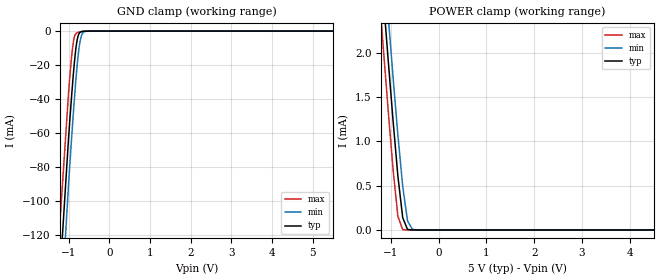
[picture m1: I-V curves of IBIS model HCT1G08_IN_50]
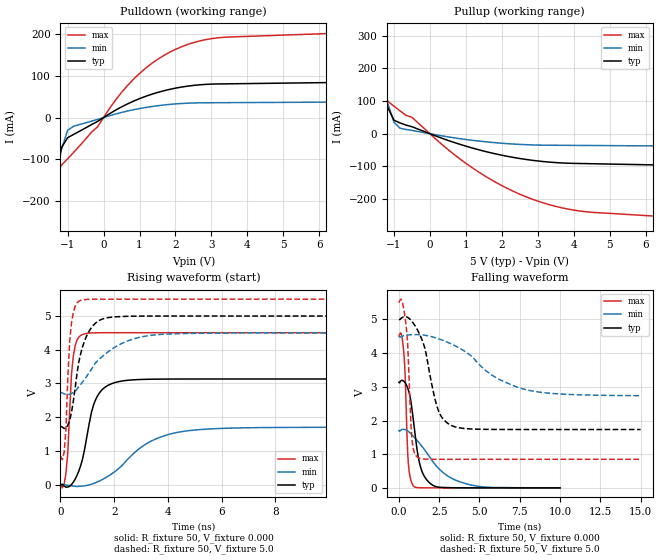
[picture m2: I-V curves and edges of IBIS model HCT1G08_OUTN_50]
| NXP Semiconductors
| Logic Products Group
| IBIS model of 74HCT1G08
| 5V 2-INPUT AND GATE
|[Packages]:
|[Package1]: TSSOP5 (GW) 5-pins Package
|[Package2]: TSSOP5 (GV) 5-pins Package
[IBIS Ver]   3.2
[File Name]   hct1g08.ibs
[File Rev]   1.0
[Date]   07-Nov-2012
[Source]   File created from simulations by LPG
   NXP Semiconductors Nijmegen
[Notes]   V1.0   Ibis model.
   Revision History
   Version Date   Author/Editor  Description
   1.0   November 2012  RRV   Initial Model
   Remarks: - IBISCHK 5.1.0 used
[Disclaimer]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
[Copyright]
   (C) Copyright 2012 NXP Semiconductors
   All rights reserved
|   Info for  TSSOP5 (GW) 5-pins Package
[Component]   74HCT1G08_GW
[Manufacturer]   NXP Semiconductors
[Package]
|   Typ   Min   Max
R_pkg   8.353E-02   8.341E-02   8.366E-02
L_pkg   1.484E-09   1.480E-09   1.486E-09
C_pkg   2.355E-13   1.892E-13   3.527E-13
[Pin] signal_name   model_name   R_pin   L_pin   C_pin
   1   B   HCT1G08_IN_50 8.357E-02 1.485E-09 2.132E-13
   2   A   HCT1G08_IN_50 8.366E-02 1.480E-09 2.311E-13
   3   GND   GND 8.354E-02 1.484E-09 1.914E-13
   4   Y   HCT1G08_OUTN_50 8.351E-02 1.486E-09 1.892E-13
   5   VCC   POWER 8.341E-02 1.486E-09 3.527E-13
|   Info for  TSSOP5 (GV) 5-pins Package
[Component]   74HCT1G08_GV
[Manufacturer]   NXP Semiconductors
[Package]
|   Typ   Min   Max
R_pkg   8.192E-02   8.186E-02   8.199E-02
L_pkg   1.305E-09   1.300E-09   1.309E-09
C_pkg   2.711E-13   2.208E-13   4.174E-13
[Pin] signal_name   model_name   R_pin   L_pin   C_pin
   1   B   HCT1G08_IN_50 8.195E-02 1.309E-09 2.208E-13
   2   A   HCT1G08_IN_50 8.199E-02 1.307E-09 2.559E-13
   3   GND   GND 8.194E-02 1.309E-09 4.174E-13
   4   Y   HCT1G08_OUTN_50 8.188E-02 1.300E-09 2.377E-13
   5   VCC   POWER 8.186E-02 1.300E-09 2.239E-13
| Models and submodels in the file (2): HCT1G08_IN_50 (Input), HCT1G08_OUTN_50 (Output)
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|   Model HCT1G08_IN_50
[Model]   HCT1G08_IN_50
Model_type   Input
Vinl = 0.8V
Vinh = 2.0V
C_comp   2.8774pF   1.2578pF   5.2328pF
[Model Spec]
| Note: The input and output voltage ratings may be exceeded if the input and
|   output current ratings are observed (please refer to the data sheet)
|   Subparameter   typ   min   max
| Thresholds
Vinl   0.8   0.8   0.8
Vinh   2.0   2.0   2.0
| Overshoot
S_overshoot_high   7.0   7.0   7.0
S_overshoot_low   -0.5   -0.5   -0.5
D_overshoot_high   7.2   7.2   7.2
D_overshoot_low   -1.3   -1.3   -1.3
D_overshoot_time   3n   3n   3n
|Ambient temperature:   25   85   -40
[Temperature Range]   35   95   -30
[Voltage Range]   5.0   4.5   5.5
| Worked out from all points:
|   GND clamp passes 1 mA (typ) near -0.73 V on its own axis
|   POWER clamp passes 1 mA (typ) near -0.92 V on its own axis
|Process Range   nominal   slow   fast
[GND_clamp]
|   voltage   I(typ)   I(min)   I(max)
-5.5V     -1.839A    -1.974A    -1.717A
-1.9V     -405mA     -453.2mA   -359.4mA
-1V       -62.81mA   -90.06mA   -36.07mA
-937.5mV  -42.01mA   -67.28mA   -18.13mA
-887.5mV  -26.77mA   -49.95mA   -7.313mA
-837.5mV  -13.86mA   -33.87mA   -2.148mA
-787.5mV  -5.045mA   -19.81mA   -915.9uA
-737.5mV  -1.287mA   -9.108mA   -551.9uA
-700mV    -465.6uA   -4.104mA   -378.7uA
-650mV    -161.3uA   -1.11mA    -204.8uA
-575mV    -48.51uA   -142.2uA   -52.35uA
5.5V      0A         0A         0A
[POWER_clamp]
|   voltage   I(typ)   I(min)   I(max)
-5.5V     34.86mA    35.34mA    34.33mA
-1.258V   3.328mA    3.828mA    2.758mA
-1.157V   2.615mA    3.117mA    2.044mA
-1.056V   1.914mA    2.414mA    1.346mA
-954.6mV  1.236mA    1.729mA    686.7uA
-853.5mV  610uA      1.075mA    154.9uA
-752.5mV  138.8uA    493uA      3.22uA
-651.5mV  5.946uA    102.1uA    26.47nA
-550.5mV  136.3nA    6.271uA    213.4pA
4.5V      4.076pA    -780.7fA   1.77fA
|   Model HCT1G08_OUTN_50
[Model]   HCT1G08_OUTN_50
Model_type   Output
Polarity   Non-Inverting
Vmeas =  1.3V
Cref  =  50e-12
Rref  =  1e6
Vref  =  0V
C_comp   2.32pF   1.86pF   2.78pF
[Model Spec]
| Note: The input and output voltage ratings may be exceeded if the input and
|   output current ratings are observed (please refer to the data sheet)
|   Subparameter   typ   min   max
| Timing Thresholds
Vmeas   1.3   1.3   1.3
|Ambient temperature:   25   85   -40
[Temperature Range]   35   95   -35
[Voltage Range]   5.0   4.5   5.5
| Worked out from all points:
|   slope of the pulldown table from 0 to 0.75 V, typ, clamps not added: 20.8 ohm
|   slope of the pullup table from 0 to 0.75 V, typ, clamps not added: 25.5 ohm
|   rising waveform, R_fixture 50, V_fixture 0.000: 20-80 % time 527ps typ, 1.63ns min, 184ps max; typ from 0 V to 3.13 V
|   rising waveform, R_fixture 50, V_fixture 5.0: 20-80 % time 479ps typ, 1.32ns min, 173ps max; typ from 1.73 V to 5 V
|   falling waveform, R_fixture 50, V_fixture 0.000: 20-80 % time 577ps typ, 1.86ns min, 199ps max; typ from 3.13 V to 0 V
|   falling waveform, R_fixture 50, V_fixture 5.0: 20-80 % time 912ps typ, 3.07ns min, 267ps max; typ from 5 V to 1.73 V
|Process Range   nominal   slow   fast
[Pulldown]
|   voltage   I(typ)   I(min)   I(max)
-5.5V     -2.373A    -2.267A    -2.616A
-1.667V   -280.9mA   -292.8mA   -272mA
-1.5V     -204.1mA   -216mA     -197.4mA
-1.333V   -131.4mA   -142mA     -136.8mA
-1.167V   -71.26mA   -74.99mA   -113.5mA
-1V       -48.22mA   -30.58mA   -98.64mA
-166.7mV  -9.396mA   -4.539mA   -22.23mA
333.3mV   17.69mA    8.49mA     41.84mA
1V        45.26mA    21.54mA    105.5mA
2.333V    75.14mA    34.39mA    174.8mA
3.333V    80.61mA    35.63mA    192.1mA
11V       88.85mA    38.92mA    215.6mA
[Pullup]
|   voltage   I(typ)   I(min)   I(max)
-5.5V     2.343A     2.275A     2.518A
-1.833V   376.8mA    392mA      363.4mA
-1.667V   297.5mA    313.2mA    283.7mA
-1.333V   145.4mA    160.5mA    138.2mA
-1.167V   78.81mA    90.31mA    99.07mA
-1V       41.58mA    35.08mA    84.33mA
-833.3mV  33.15mA    16.93mA    70.32mA
-500mV    21.48mA    10.24mA    50.38mA
1.333V    -48.38mA   -22.07mA   -115.7mA
3V        -83.4mA    -34.69mA   -206.4mA
4.5V      -91.87mA   -36.04mA   -240.7mA
11V       -105.3mA   -40.62mA   -284.2mA
[Ramp]
| variable   typ   min   max
dV/dt_r  1.8800E+00/5.2612E-10  1.0207E+00/1.6255E-09  2.7029E+00/1.8002E-10
dV/dt_f  1.8800E+00/5.7700E-10  1.0209E+00/1.8619E-09  2.7029E+00/1.9925E-10
R_load = 50
[Rising Waveform]
R_fixture   = 50
V_fixture   = 0.000
V_fixture_min = 0.000
V_fixture_max = 0.000
| time   V(typ)   V(min)   V(max)
0s        219.7pV    647pV      69.87pV
204.6ps   -72.98mV   -7.331mV   341.1mV
272.7ps   -68.68mV   -15.83mV   938.4mV
409.1ps   3.237mV    -30.83mV   3.244V
477.3ps   73.93mV    -39.65mV   3.806V
818.2ps   747.2mV    -40.36mV   4.451V
1.295ns   2.495V     57.11mV    4.502V
2.182ns   3.057V     490.4mV    4.505V
4.8ns     3.133V     1.604V     4.505V
15ns      3.133V     1.702V     4.505V
[Rising Waveform]
R_fixture   = 50
V_fixture   = 5.0
V_fixture_min = 4.5
V_fixture_max = 5.5
| time   V(typ)   V(min)   V(max)
0s        1.733V     2.732V     848mV
136.4ps   1.666V     2.691V     955.6mV
204.6ps   1.67V      2.675V     1.651V
340.9ps   1.905V     2.681V     4.225V
409.1ps   2.131V     2.701V     4.779V
545.5ps   2.854V     2.775V     5.283V
750ps     3.873V     2.969V     5.461V
1.432ns   4.862V     3.711V     5.5V
3.341ns   4.998V     4.425V     5.5V
15ns      5V         4.5V       5.5V
[Falling Waveform]
R_fixture   = 50
V_fixture   = 0.000
V_fixture_min = 0.000
V_fixture_max = 0.000
| time   V(typ)   V(min)   V(max)
0s        3.133V     1.702V     4.505V
272.7ps   3.179V     1.738V     4.18V
363.6ps   3.135V     1.731V     3.619V
500ps     3.022V     1.704V     1.604V
590.9ps   2.903V     1.675V     696.8mV
909.1ps   1.972V     1.524V     51.95mV
1.364ns   589mV      1.273V     3.088mV
2.182ns   59.54mV    732.3mV    60.87uV
4.6ns     504.3uV    72.62mV    500nV
10ns      1.28uV     809.6uV    57.32nV
[Falling Waveform]
R_fixture   = 50
V_fixture   = 5.0
V_fixture_min = 4.5
V_fixture_max = 5.5
| time   V(typ)   V(min)   V(max)
0s        5V         4.5V       5.5V
409.1ps   5.081V     4.53V      4.973V
545.5ps   5.061V     4.539V     4.279V
818.2ps   4.937V     4.55V      1.419V
1.159ns   4.684V     4.551V     909.6mV
1.636ns   4.101V     4.53V      853.6mV
2.455ns   2.293V     4.429V     848.2mV
3.273ns   1.849V     4.269V     848mV
7.895ns   1.733V     2.914V     848mV
15ns      1.733V     2.738V     848mV
